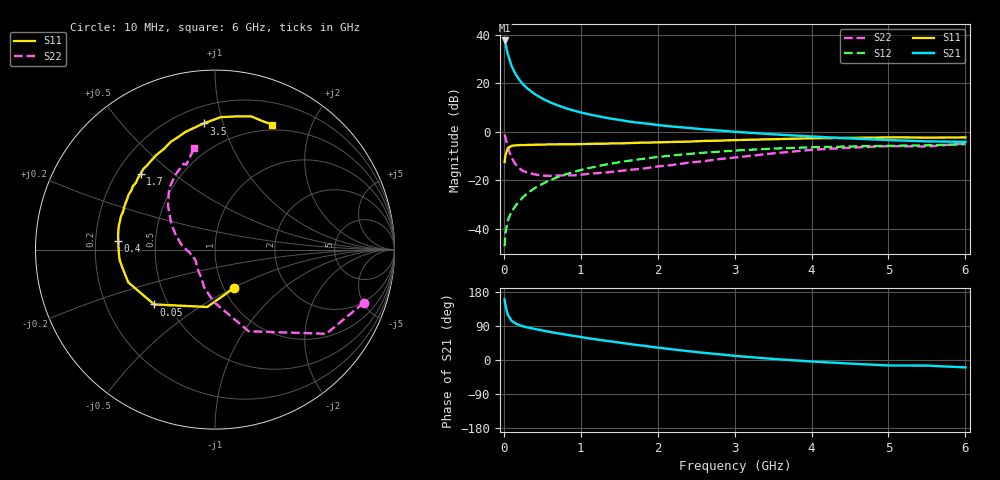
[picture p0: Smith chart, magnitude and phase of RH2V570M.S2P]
! SIEMENS Small Signal Semiconductors
! BFR106
! Si NPN RF Bipolar Junction Transistor in SOT23
! VCE = 2.5 V  IC = 70 mA
! Common Emitter S-Parameters:  August  1996
# GHz  S  MA  R  50
!  f  S11  S21  S12  S22
! GHz  MAG  ANG  MAG  ANG  MAG  ANG  MAG  ANG
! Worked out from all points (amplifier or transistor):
!   36 points, 10 MHz to 6 GHz, reference 50 ohm
!   highest |S21| = 37.7 dB at 10 MHz (marker M1)
!   |S21| within 3 dB of that: start of sweep to 32.54 MHz
!   unconditionally stable (mu >= 1): 195.1 MHz to 2.575 GHz; 5.275 GHz to end of sweep
!   at 250 MHz: K = 1.04, MAG = 22.0 dB, |S12| = -26.9 dB
!   at 1.4 GHz: K = 1.06, MAG = 7.7 dB, |S12| = -13.1 dB
!   at 6 GHz: K = 1.00, MAG = 0.1 dB, |S12| = -5.1 dB
!   S11 on the Smith chart (normalised r, x): 10 MHz: 1.11, -0.51; 50 MHz: 0.42, -0.32; 400 MHz: 0.30, +0.04; 1.7 GHz: 0.30, +0.39; 3.5 GHz: 0.31, +0.86; 6 GHz: 0.43, +1.47
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0.01  0.2391 -63.8  76.65 160.3  0.0044 78.7  0.8799 -19.7
0.02  0.3225 -97.7  66.62 145.1  0.0081 69.1  0.7775 -37.1
0.05  0.4565 -138.0  40.78 119.6  0.0148 60.5  0.4922 -67.6
0.1  0.5165 -159.3  23.03 103.9  0.0225 63.5  0.2909 -91.5
0.15  0.5256 -168.9  15.69 96.6  0.0296 67.0  0.2179 -106.2
0.2  0.5344 -173.7  11.94 92.3  0.0371 70.3  0.1773 -115.0
0.25  0.5358 -177.3  9.551 88.8  0.045 70.9  0.1561 -124.6
0.3  0.5371 179.5  7.998 86.3  0.0532 72.2  0.1464 -130.5
0.4  0.5421 174.8  6.054 82.0  0.0691 72.7  0.1325 -140.8
0.5  0.5466 170.8  4.86 77.9  0.0843 72.3  0.1254 -147.9
0.6  0.5514 166.8  4.078 74.1  0.1008 71.6  0.1241 -152.3
0.7  0.5529 163.7  3.523 70.4  0.1166 70.5  0.126 -156.7
0.9  0.5547 157.5  2.773 63.9  0.1481 67.7  0.1266 -164.4
1.1  0.5639 150.5  2.309 57.3  0.1783 64.7  0.1365 -168.9
1.3  0.5706 144.8  1.987 51.5  0.208 61.5  0.1441 -174.1
1.7  0.5922 134.4  1.578 40.3  0.2637 55.0  0.1684 176.4
2.2  0.6198 122.0  1.284 27.9  0.3275 46.5  0.2081 165.3
3  0.6759 104.2  1.006 11.0  0.4112 33.4  0.2952 146.8
3.5  0.7057 95.2  0.891 2.8  0.4521 25.7  0.3603 136.7
4.5  0.7519 80.8  0.731 -9.5  0.4999 11.3  0.4712 118.0
5.5  0.763 69.2  0.637 -14.8  0.5273 2.5  0.4993 108.7
6  0.7664 65.4  0.623 -19.5  0.5558 -4.3  0.5769 101.6
